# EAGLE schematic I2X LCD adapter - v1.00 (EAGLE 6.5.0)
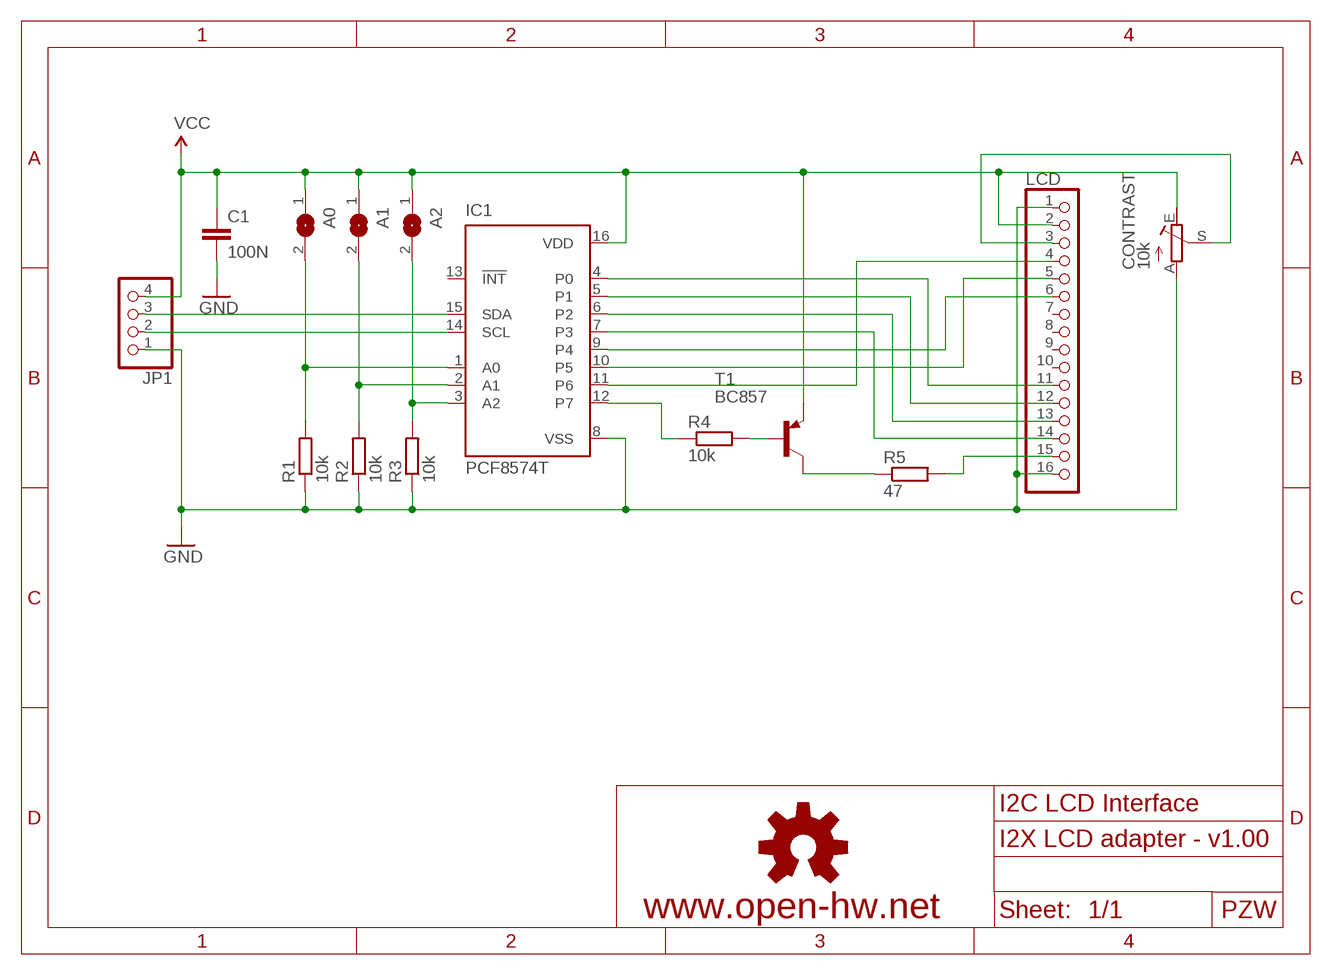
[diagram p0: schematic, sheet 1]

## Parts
A0  SJ  [SJ]
A1  SJ  [SJ]
A2  SJ  [SJ]
C1  100N  C-EUC0805  [C0805]
CONTRAST  10k  PCT6  [CT6]
IC1  PCF8574T  [SO16W]
JP1  PINHD-1X4/90  [1X04/90]
LCD  PINHD-1X16  [1X16]
R1  10k  R-EU_R0805  [R0805]
R2  10k  R-EU_R0805  [R0805]
R3  10k  R-EU_R0805  [R0805]
R4  10k  R-EU_R0805  [R0805]
R5  47  R-EU_R0805  [R0805]
T1  BC857  BC857BSMD  [SOT23-BEC]

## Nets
GND: C1.2 CONTRAST.A IC1.8(VSS) JP1.1 LCD.1 LCD.16 R1.1 R2.1 R3.1
N$1: IC1.14(SCL) JP1.2
N$2: IC1.15(SDA) JP1.3
N$3: A0.2 IC1.1(A0) R1.2
N$4: A1.2 IC1.2(A1) R2.2
N$5: A2.2 IC1.3(A2) R3.2
N$6: IC1.12(P7) R4.1
N$7: R5.1 T1.C
N$8: R4.2 T1.B
N$9: LCD.15 R5.2
N$10: CONTRAST.S LCD.3
N$11: IC1.4(P0) LCD.11
N$12: IC1.5(P1) LCD.12
N$13: IC1.6(P2) LCD.13
N$14: IC1.7(P3) LCD.14
N$15: IC1.9(P4) LCD.6
N$16: IC1.10(P5) LCD.5
N$17: IC1.11(P6) LCD.4
VCC: A0.1 A1.1 A2.1 C1.1 CONTRAST.E IC1.16(VDD) JP1.4 LCD.2 T1.E
Unconnected: IC1.13(!INT) LCD.7 LCD.8 LCD.9 LCD.10

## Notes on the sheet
- I2C LCD Interface
- PZW

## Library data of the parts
A0 A1 A2 = jumper:SJ: SMD solder JUMPER
C1 = rcl:C-EU: CAPACITOR, European symbol
CONTRAST = work:P
IC1 = micro-philips:PCF8574: I2C-Bus Remote 8-bit I/O expander http://www.semiconductors.philips.com/acrobat_download/datasheets/PCF8574_4.pdf; MPN: PCF8574T/3,512; OC_FARNELL: 1201255; OC_NEWARK: 70R6870
JP1 = pinhead:PINHD-1X4: PIN HEADER
LCD = pinhead:PINHD-1X16: PIN HEADER
R1-R5 = rcl:R-EU_: RESISTOR, European symbol
T1 = transistor-pnp:BC857*: PNP Transistror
